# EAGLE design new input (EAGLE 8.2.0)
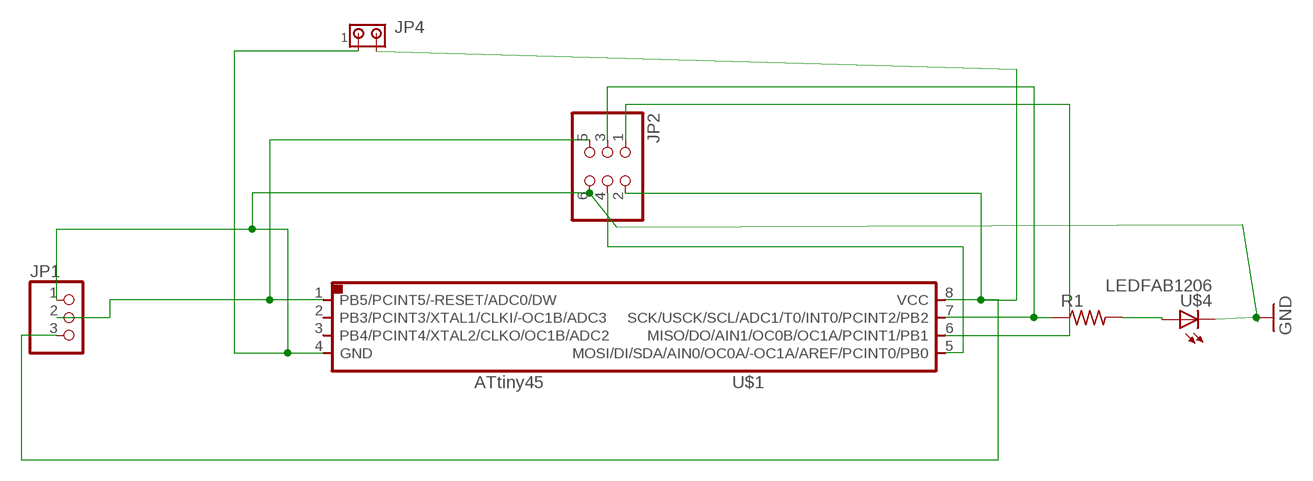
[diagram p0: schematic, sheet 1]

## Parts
JP1  PINHD-1X3  [1X03]
JP2  PINHD-2X3-SMD  [2X03SMD]
JP4  MTA02-156  [1X2MTA]
R1  RES-US1206  [R1206]
U$1  ATTINY45SI  [SOIC8]
U$4  LEDFAB1206  [LED1206FAB]

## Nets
GND: JP1.1 JP2.6 JP4.1 U$1.4(GND) U$4.2(C)
N$2: JP1.3 JP2.2 JP4.2 U$1.8(VCC)
N$3: JP1.2 JP2.5 U$1.1(PB5/PCINT5/-RESET/ADC0/DW)
N$4: JP2.4 U$1.5(MOSI/DI/SDA/AIN0/OC0A/-OC1A/AREF/PCINT0/PB0)
N$5: JP2.3 R1.1 U$1.7(SCK/USCK/SCL/ADC1/T0/INT0/PCINT2/PB2)
N$6: JP2.1 U$1.6(MISO/DO/AIN1/OC0B/OC1A/PCINT1/PB1)
N$7: R1.2 U$4.1(A)
Unconnected: U$1.2(PB3/PCINT3/XTAL1/CLKI/-OC1B/ADC3) U$1.3(PB4/PCINT4/XTAL2/CLKO/OC1B/ADC2)

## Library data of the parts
JP1 = pinhead:PINHD-1X3: PIN HEADER
JP2 = fab:PINHD-2X3-SMD: PIN HEADER
JP4 = con-amp:MTA02-156: AMP connector
R1 = fab:RES-US: Resistor (US Symbol)
U$1 = fab:ATTINY45
U$4 = fab:LED: LED

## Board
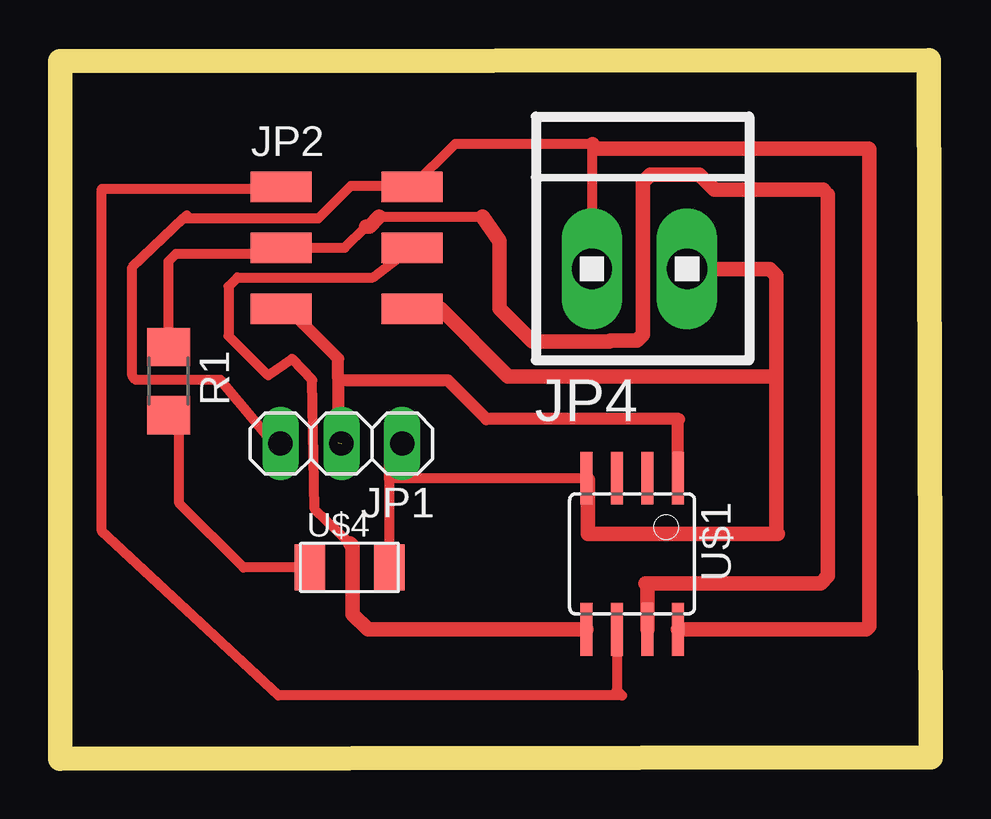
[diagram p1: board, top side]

Size 36.31 x 29.13 mm. Coordinates in mm from the lower left corner, seen from the top.
Outline: 0,0 36.31,0.06 36.21,29.13 0.02,29.08 0,0
Copper layers (1*16): Top 0.035mm / dielectric 1.5mm / Bottom 0.035mm
Design rules "default *": minimum track width 6mil, minimum drill 0.35mm, track to track 8mil, track to pad 8mil, pad to pad 6mil, via to via 6mil, smd to smd 6mil, copper to edge 40mil, drill to drill 6mil, minimum pad ring 10mil, minimum via ring 8mil, stop-mask expansion 8mil, vias tented up to drill 0mil, thermal gap 10mil

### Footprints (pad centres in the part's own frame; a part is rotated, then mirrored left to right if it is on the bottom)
1X03 = drill 1.016 long: 1 -2.54,0; 2 0,0; 3 2.54,0
2X03SMD = smd 2.54 x 1.27: 1 -2.54,2.54; 2 2.92,2.54; 3 -2.54,0; 4 2.92,0; 5 -2.54,-2.54; 6 2.92,-2.54
1X2MTA = drill 1.676 long: 1 1.981,0; 2 -1.981,0
R1206 = smd 1.6 x 1.803: 1 -1.422,0; 2 1.422,0
SOIC8 = smd 0.5 x 2.2: 1 -1.905,-3.154; 2 -0.645,-3.154; 3 0.625,-3.154; 4 1.895,-3.154; 5 1.905,3.154; 6 0.635,3.154; 7 -0.635,3.154; 8 -1.905,3.154
LED1206FAB = smd 1.27 x 1.905: 1 -1.651,0; 2 1.651,0

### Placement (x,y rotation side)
JP1  11.73,13.14 180 top
JP2  11.76,21.3 0 top
JP4  24.16,20.42 0 top
R1  4.53,15.74 270 top
U$1  23.85,8.54 180 top
U$4  12.07,7.97 0 top

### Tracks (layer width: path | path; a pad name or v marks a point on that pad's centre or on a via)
GND
  Top 0.406: 13.72,11.62 U$4.2 | 13.72,11.62 13.72,12.59 JP1.1 | U$1.4 13.79,11.69 13.72,11.62
  Top 0.61: JP4.1 29.59,20.42 29.86,20.15 29.86,15.88 | 29.86,15.88 29.86,9.43 29.92,9.37 22.02,9.37 22.02,11.63 U$1.4 | JP2.6 15.86,18.76 18.68,15.94 29.8,15.94 29.86,15.88
N$2
  Top 0.406: JP4.2 22.18,25.61 22.2,25.63 16.47,25.63 JP2.2 14.63,23.89 12.13,23.89 10.78,22.54 5.16,22.54 | JP1.3 8.85,13.22 6.69,15.79 3.16,15.79 3.02,15.97 3.02,20.49 5.16,22.54 | 5.16,22.54 5.29,22.66
  Top 0.61: U$1.8 33.61,5.39 33.74,5.52 33.74,25.41 33.72,25.43 22.4,25.43 22.2,25.63
N$3  (1 unrouted)
  Top 0.508: JP2.5 9.52,18.76 11.6,16.68 11.6,15.84 | 11.6,15.84 11.6,13.18 12.14,12.64 | U$1.1 25.75,14.1 25.82,14.16 17.78,14.16 16.17,15.77 11.67,15.77 11.6,15.84
N$4
  Top 0.406: 12.1,8.97 10.62,10.4 10.52,15.78 9.67,16.67 8.68,15.98 7.03,17.63 7.03,19.69 7.4,20.06 13.05,20.06 JP2.4
  Top 0.61: U$1.5 12.83,5.39 12.2,6.02 12.2,8.87 12.1,8.97
N$5
  Top 0.406: R1.1 4.53,20.74 4.84,21.05 8.97,21.05 JP2.3 | 9.74,21.11 9.41,21.11 JP2.3 | JP2.3 11.87,21.3 12.76,22.19 12.91,22.34 | 13.3,22.59 17.62,22.59
  Top 0.61: U$1.7 24.49,7.24 24.41,7.31 31.71,7.31 32.02,7.62 32.02,23.52 31.82,23.72 27.28,23.72 26.66,24.34 24.61,24.34 24.3,24.03 24.3,17.68 24.05,17.43 22.94,17.43 22.91,17.4 19.7,17.4 18.33,18.77 18.33,21.57 17.62,22.59 | 12.76,22.19 12.9,22.19 13.3,22.59
N$6
  Top 0.406: U$1.6 23.21,2.86 23.43,2.64 9.11,2.64 1.74,9.49 1.74,23.76 9.14,23.76 JP2.1
N$7
  Top 0.406: U$4.1 7.65,7.97 4.97,10.65 4.97,13.88 R1.2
